FUNCTION_BLOCK Axis_PTP_Ex2 EXTENDS Axis_PTP_Ex
VAR_INPUT
END_VAR
VAR_OUTPUT
END_VAR
VAR
END_VAR

;

METHOD M_Home : BOOL
VAR_INPUT
	Execute:BOOL;
END_VAR
VAR_STAT
	mcHome:FB_Home_ByLimit;
END_VAR
CASE PARA.HomingMode OF 	
0:
	mcHome(
		Axis:= REF, 
		Execute:= Execute, 
		PosLimit:= DrvIn.Limit_Pos, 
		NegLimit:= DrvIn.Limit_Neg, 
		Position:= PARA.RefPos,
		bCalibrationCam:= DrvIn.HomeSensor);
1:	
	SUPER^.M_Home(Execute:= Execute);

END_CASE
END_METHOD

END_FUNCTION_BLOCK
